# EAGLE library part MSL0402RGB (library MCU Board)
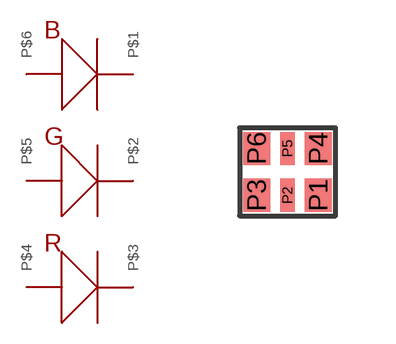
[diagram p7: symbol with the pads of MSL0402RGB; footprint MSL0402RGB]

Designator prefix D

## MSL0402RGB  [MSL0402RGB]
P1  P$1
P2  P$2
P3  P$3
P4  P$4
P5  P$5
P6  P$6

## Footprint MSL0402RGB (pad centres in mm)
smd 0.67 x 0.83: P1 0.77,-0.585; P3 -0.77,-0.585; P4 0.77,0.585; P6 -0.77,0.585
smd 0.37 x 0.83: P2 0,-0.585; P5 0,0.585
